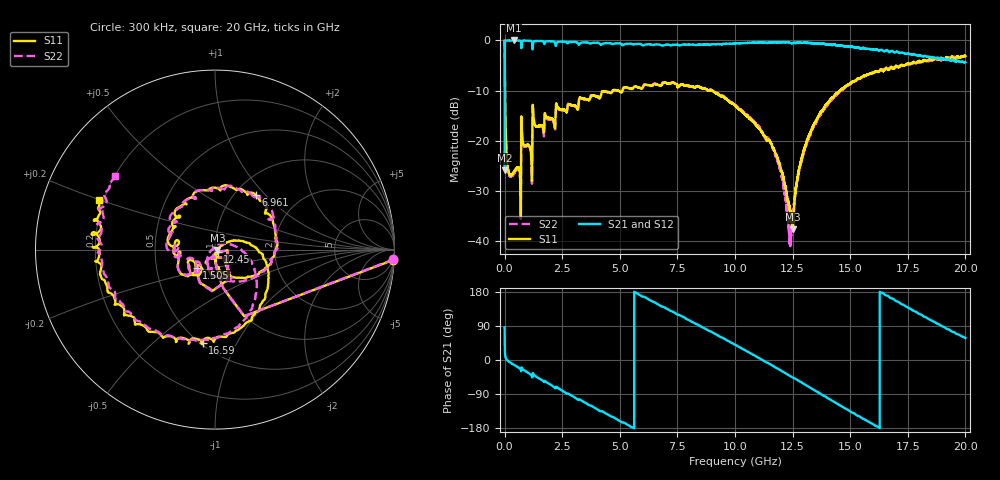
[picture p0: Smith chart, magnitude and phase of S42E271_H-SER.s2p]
! Created Wed Nov 25 22:09:03 2020
# khz S ma R 50
! 2 Port Network Data from SP1.SP block
! freq  magS11  angS11  magS21  angS21  magS12  angS12  magS22  angS22
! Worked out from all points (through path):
!   20001 points, 300 kHz to 20 GHz, reference 50 ohm
!   highest |S21| = -0.02 dB at 392.3 MHz (marker M1); lowest = -25.8 dB at 300 kHz (marker M2)
!   group delay of S21, straight-line fit = 92.6 ps
!   lowest |S11| = -37.6 dB at 12.5 GHz (marker M3), VSWR 1.03, Z = 51.3 - j0.229 ohm
!   |S11| at or under -10 dB: 17.73 MHz to 4.692 GHz (4.674 GHz wide, 198 % of centre); 4.929 GHz to 5.116 GHz (186.6 MHz wide, 3.72 % of centre); 9.015 GHz to 14.56 GHz (5.543 GHz wide, 47 % of centre)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
!   |S22| runs from -40.9 to 0.0 dB; largest |S21 - S12| = 0.017
!   S11 on the Smith chart (normalised r, x): 300 kHz: 4, -34; 1.505 GHz: 0.80, -0.16; 6.961 GHz: 1.24, +0.88; 12.45 GHz: 1.03, -0.02; 16.59 GHz: 0.51, -0.74; 20 GHz: 0.18, +0.20
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300  0.9933 -3.4  0.05124 86.2  0.05073 86.1  0.9954 -3.2
103300  0.06623 -88.4  0.9948 -0.2  0.9952 -0.2  0.06552 -88.5
199300  0.04721 -94.0  0.9959 -5.0  0.9964 -5.0  0.04596 -93.9
392300  0.04888 -101.4  0.9972 -12.4  0.997 -12.3  0.04661 -100.7
816300  0.09262 -115.5  0.9923 -25.9  0.9915 -25.9  0.09053 -115.9
1505300  0.1426 -135.4  0.9851 -49.0  0.985 -49.0  0.1389 -143.3
3334300  0.265 160.4  0.9491 -106.9  0.9492 -106.9  0.2633 167.0
4961300  0.3127 111.2  0.9311 -159.8  0.9319 -159.7  0.312 111.9
6667300  0.3609 60.8  0.91 146.4  0.909 146.3  0.3631 54.1
6961300  0.3801 53.4  0.9003 138.0  0.9022 137.9  0.3827 45.0
8496300  0.3407 1.0  0.9083 89.2  0.9092 89.3  0.3386 -0.8
1.00003e7  0.2246 -44.8  0.9329 40.3  0.931 40.3  0.2272 -51.1
1.15213e7  0.098 -81.4  0.9533 -11.1  0.9532 -11.1  0.09869 -113.2
1.24533e7  0.01813 -38.2  0.9335 -44.6  0.9345 -44.7  0.01302 140.6
1.25013e7  0.01323 -9.7  0.938 -45.7  0.939 -45.7  0.01729 109.0
1.28053e7  0.05533 32.0  0.9496 -56.2  0.9464 -56.2  0.05375 38.2
1.33343e7  0.1302 22.2  0.9408 -75.6  0.94 -75.6  0.1275 5.3
1.50303e7  0.3759 -41.6  0.8614 -136.9  0.8637 -136.9  0.3729 -55.6
1.65873e7  0.5258 -97.6  0.8002 170.0  0.7906 170.2  0.5165 -102.5
1.66673e7  0.5084 -102.3  0.7713 167.9  0.775 167.1  0.5266 -105.4
1.82553e7  0.6294 -151.8  0.6994 113.2  0.6904 113.8  0.6239 -160.1
2e7  0.699 157.0  0.6056 57.8  0.6051 58.1  0.6966 143.3
